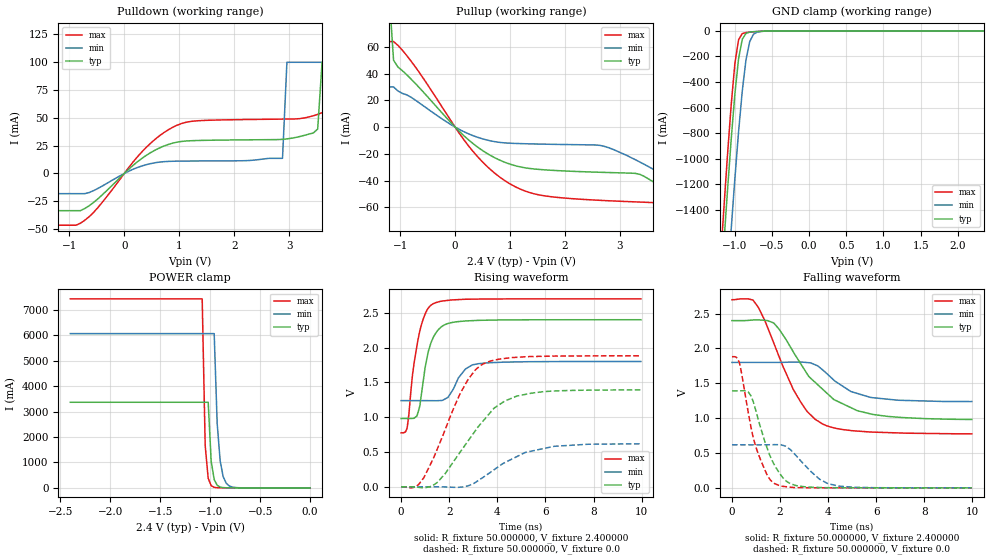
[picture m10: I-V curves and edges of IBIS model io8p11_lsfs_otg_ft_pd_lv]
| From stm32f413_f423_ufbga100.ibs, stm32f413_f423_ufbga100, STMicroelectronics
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|   Model io8p11_lsfs_otg_ft_pd_lv
[Model]  io8p11_lsfs_otg_ft_pd_lv
Model_type I/O
Polarity   Non-Inverting
Enable   Active-Low
Vinl =   0.720000V
Vinh =   1.680000V
Vmeas =  1.200000V
Cref =   30.000000pF
Rref =   100.000000M
Vref =   0.0V
C_comp   7.971100pF   7.737700pF   8.264100pF
[Temperature Range]   25.000000   0.125000k   -40.000000
[Pullup Reference]   2.400000V   1.800000V   2.700000V
[Pulldown Reference]   0.0V   0.0V   0.0V
[POWER Clamp Reference]   2.400000V   1.800000V   2.700000V
[GND Clamp Reference]   0.0V   0.0V   0.0V
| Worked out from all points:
|   slope of the pulldown table from 0 to 0.36 V, typ, clamps not added: 24.1 ohm
|   slope of the pullup table from 0 to 0.36 V, typ, clamps not added: 26.8 ohm
|   GND clamp passes 1 mA (typ) near -0.52 V on its own axis
|   POWER clamp passes 1 mA (typ) near -0.81 V on its own axis
|   rising waveform, R_fixture 50.000000, V_fixture 2.400000: 20-80 % time 481ps typ, 591ps min, 481ps max; typ from 0.981 V to 2.4 V
|   rising waveform, R_fixture 50.000000, V_fixture 0.0: 20-80 % time 1.81ns typ, 1.82ns min, 1.43ns max; typ from 0 V to 1.39 V
|   falling waveform, R_fixture 50.000000, V_fixture 2.400000: 20-80 % time 1.98ns typ, 1.46ns min, 1.53ns max; typ from 2.4 V to 0.981 V
|   falling waveform, R_fixture 50.000000, V_fixture 0.0: 20-80 % time 862ps typ, 1.06ns min, 753ps max; typ from 1.39 V to 0 V
[Pulldown]
|Voltage   I(typ)   I(min)   I(max)
-2.4V     -33.44mA   -18.12mA   -46.52mA
-800mV    -33.44mA   -18.12mA   -44.78mA
1.04V     28.81mA    11.14mA    44.91mA
2.88V     30.7mA     13.64mA    48.89mA
2.96V     31.11mA    100mA      48.94mA
3.52V     40mA       100mA      53.15mA
3.6V      100mA      100mA      54.65mA
3.92V     100mA      100mA      60mA
4V        100mA      100mA      100mA
4.4V      100mA      100mA      100mA
4.48V     100mA      100mA      1A
4.8V      100mA      100mA      1A
[Pullup]
|Voltage   I(typ)   I(min)   I(max)
-2.4V     100mA      1A         100mA
-1.6V     100mA      1A         100mA
-1.52V    100mA      30mA       100mA
-1.28V    100mA      30mA       100mA
-1.2V     100mA      30mA       64mA
-1.12V    50mA       30mA       64mA
-1.04V    44.9mA     27mA       61.1mA
320mV     -12.14mA   -6.322mA   -17.91mA
1.12V     -29.18mA   -12.28mA   -45.16mA
3.36V     -35.34mA   -26.1mA    -56.1mA
4V        -52.4mA    -42mA      -67mA
4.72V     -74mA      -42mA      -94.8mA
[GND_clamp]
|Voltage   I(typ)   I(min)   I(max)
-2.4V     -9.765A    -9.942A    -9.572A
-1.2V     -2.124A    -2.851A    -1.855A
-1.15V    -1.682A    -2.408A    -1.408A
-1.1V     -1.256A    -1.975A    -979.8mA
-1.05V    -854.9mA   -1.557A    -584.5mA
-1V       -496.5mA   -1.158A    -257.5mA
-950mV    -217.7mA   -789.7mA   -69.53mA
-900mV    -65.58mA   -469.8mA   -21.52mA
-850mV    -19.65mA   -226.4mA   -13.58mA
-800mV    -9.766mA   -84.22mA   -10.49mA
-700mV    -4.935mA   -9.894mA   -5.821mA
2.35V     58.09uA    37.92uA    67.25uA
[POWER_clamp]
|Voltage   I(typ)   I(min)   I(max)
-2.4V     3.365A     6.064A     7.43A
-1.08V    3.365A     6.064A     7.43A
-1.05V    3.365A     6.064A     1.669A
-1.02V    3.365A     6.064A     375mA
-990mV    1.047A     6.064A     84.24mA
-960mV    325.6mA    6.064A     18.93mA
-930mV    101.3mA    2.529A     4.252mA
-900mV    31.51mA    1.055A     955.2uA
-870mV    9.804mA    440.1mA    214.6uA
-840mV    3.05mA     183.6mA    74uA
-720mV    28.58uA    5.557mA    74uA
0V        0A         0A         0A
[Ramp]
| variable   typ   min   max
dV/dt_r  0.83394/1.81035n   0.36905/1.81039n   1.12782/1.42718n
dV/dt_f  0.84823/1.98187n   0.33528/1.46376n   1.15315/1.52996n
R_load = 50.000000
[Rising Waveform]
R_fixture= 50.000000
V_fixture= 2.400000
V_fixture_min= 1.800000
V_fixture_max= 2.700000
|time   V(typ)   V(min)   V(max)
0s        980.6mV    1.238V     774.6mV
260.3ps   980.3mV    1.238V     872.3mV
480.5ps   982.3mV    1.238V     1.63V
660.7ps   1.021V     1.238V     2.032V
780.8ps   1.173V     1.238V     2.244V
981ps     1.673V     1.238V     2.467V
1.321ns   2.134V     1.236V     2.626V
1.942ns   2.344V     1.282V     2.677V
2.963ns   2.386V     1.751V     2.695V
9.97ns    2.399V     1.799V     2.699V
[Rising Waveform]
R_fixture= 50.000000
V_fixture= 0.0
V_fixture_min= 0.0
V_fixture_max= 0.0
|time   V(typ)   V(min)   V(max)
0s        15.64uV    7.253uV    -171.9uV
600.6ps   -3.263mV   4.316uV    1.327mV
940.9ps   -12.43mV   24.09uV    129.4mV
1.502ns   61.98mV    -112.4uV   541.2mV
2.462ns   502.5mV    -5.528mV   1.344V
3.083ns   804.2mV    61.71mV    1.678V
3.383ns   935.4mV    130mV      1.759V
4.304ns   1.23V      346.5mV    1.843V
5.405ns   1.344V     511.2mV    1.87V
9.97ns    1.391V     617.3mV    1.881V
[Falling Waveform]
R_fixture= 50.000000
V_fixture= 2.400000
V_fixture_min= 1.800000
V_fixture_max= 2.700000
|time   V(typ)   V(min)   V(max)
0s        2.399V     1.799V     2.699V
880.9ps   2.408V     1.799V     2.691V
1.361ns   2.403V     1.799V     2.403V
1.742ns   2.363V     1.799V     2.074V
2.823ns   1.799V     1.804V     1.251V
3.203ns   1.594V     1.795V     1.069V
3.764ns   1.416V     1.693V     916.6mV
4.925ns   1.154V     1.386V     822.8mV
5.766ns   1.061V     1.297V     800.6mV
9.97ns    980.6mV    1.238V     774.6mV
[Falling Waveform]
R_fixture= 50.000000
V_fixture= 0.0
V_fixture_min= 0.0
V_fixture_max= 0.0
|time   V(typ)   V(min)   V(max)
0s        1.391V     617.3mV    1.881V
320.3ps   1.392V     617.3mV    1.779V
780.8ps   1.324V     617.2mV    885.8mV
981ps     1.121V     617mV      600.1mV
1.221ns   828.3mV    617mV      375.7mV
1.762ns   329.9mV    619.7mV    62.67mV
2.482ns   52.87mV    529.6mV    7.515mV
3.644ns   5.078mV    123.1mV    226.5uV
4.424ns   1.454mV    26.19mV    238.4uV
9.97ns    15.64uV    7.253uV    -171.9uV
